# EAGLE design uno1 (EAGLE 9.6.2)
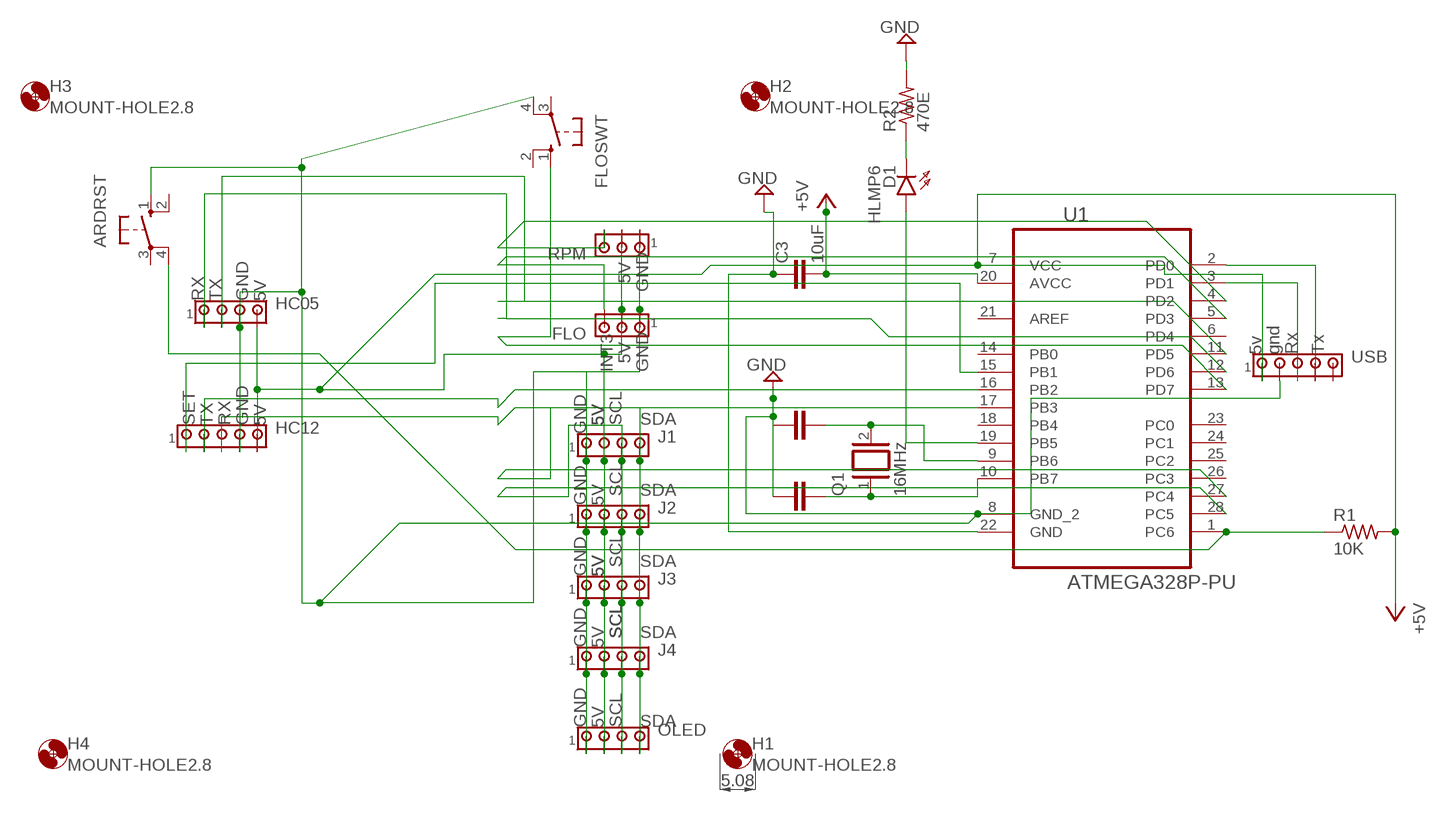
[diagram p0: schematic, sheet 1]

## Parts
ARDRST  10-XX  [B3F-10XX]
C3  10uF  C2.5/2  [C2.5-2]
D1  HLMP6  [HLMP6]
FLO  MTA03-100  [10X03MTA]
FLOSWT  10-XX  [B3F-10XX]
H1  MOUNT-HOLE2.8  [2,8]
H2  MOUNT-HOLE2.8  [2,8]
H3  MOUNT-HOLE2.8  [2,8]
H4  MOUNT-HOLE2.8  [2,8]
HC05  MTA04-100  [10X04MTA]
HC12  MTA05-100  [10X05MTA]
J1  MTA04-100  [10X04MTA]
J2  MTA04-100  [10X04MTA]
J3  MTA04-100  [10X04MTA]
J4  MTA04-100  [10X04MTA]
OLED  MTA04-100  [10X04MTA]
Q1  16MHz  XTAL  [Q]
R1  10K  R-US_0204/5  [0204/5]
R2  470E  R-US_0204/5  [0204/5]
RPM  MTA03-100  [10X03MTA]
U1  ATMEGA328P-PU  [DIP254P762X457-28]
USB  MTA05-100  [10X05MTA]

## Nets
GND: ARDRST.1(S) C3.1 FLO.1 FLOSWT.4(P1) HC05.3 HC12.4 J1.1 J2.1 J3.1 J4.1 OLED.1 R2.2 RPM.1 U1.8(GND_2) U1.22(GND) USB.2
N$1: J1.3 J2.3 J3.3 J4.3 OLED.3 U1.28(PC5)
N$2: J1.4 J2.4 J3.4 J4.4 OLED.4 U1.27(PC4)
N$3: U1.2(PD0) USB.4
N$4: HC12.1 U1.15(PB1)
N$5: U1.3(PD1) USB.3
N$6: FLO.3 U1.5(PD3)
N$7: FLOSWT.1(S) U1.13(PD7)
N$8: HC05.2 U1.11(PD5)
N$9: HC05.1 U1.12(PD6)
N$10: HC12.2 U1.16(PB2)
N$11: HC12.3 U1.17(PB3)
N$13: ARDRST.4(P1) R1.1 U1.1(PC6)
N$14: RPM.3 U1.4(PD2)
N$15: Q1.2 U1.9(PB6)
N$16: Q1.1 U1.10(PB7)
N$21: D1.A U1.19(PB5)
N$22: D1.K R2.1
VCC: C3.2 FLO.2 HC05.4 HC12.5 J1.2 J2.2 J3.2 J4.2 OLED.2 R1.2 RPM.2 U1.7(VCC) U1.20(AVCC) USB.1 ; supply symbol labelled +5V
Unconnected: ARDRST.2(S1) ARDRST.3(P) FLOSWT.2(S1) FLOSWT.3(P) U1.6(PD4) U1.14(PB0) U1.18(PB4) U1.21(AREF) U1.23(PC0) U1.24(PC1) U1.25(PC2) U1.26(PC3) USB.5

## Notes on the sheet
- 5V
- GND
- RX | TX | GND | 5V
- 5v | gnd | Rx | Tx
- 5V
- INT3 | GND
- SET | TX | RX | GND | 5V | 5V | 5V | 5V | SCL | SDA
- GND
- SCL | SDA
- GND | 5V
- SCL | SDA
- GND | 5V | 5V
- SCL | SCL | SCL | SDA
- GND | 5V
- GND | 5V | SCL | SDA

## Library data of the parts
ARDRST FLOSWT = switch-omron:10-XX: OMRON SWITCH; MPN: B3F-1000; OC_FARNELL: 176432; OC_NEWARK: 36M3542
C3 = capacitor-wima:C: CAPACITOR
D1 = display-hp:HLMP6: LED; MF: AGILENT TECHNOLOGIES; MPN: HLMP-6500; OC_FARNELL: 1652490; OC_NEWARK: 40K0088
FLO RPM = con-amp:MTA03-100: AMP connector
H1-H4 = holes:MOUNT-HOLE: MOUNTING HOLE with drill center marker
HC05 J1-J4 OLED = con-amp:MTA04-100: AMP connector
HC12 USB = con-amp:MTA05-100: AMP connector
Q1 = special:XTAL: CRYSTAL
R1 R2 = rcl:R-US_: RESISTOR, American symbol; SPICEPREFIX: R
U1 = Atmel_By_element14_Batch_1-00:ATMEGA328P-PU: 8-bit Microcontroller with In-System Programmable Flash; MPN: ATMEGA328P-PU; OC_FARNELL: 1715487; OC_NEWARK: 15R0268; PACKAGE: PDIP-28; SUPPLIER: Atmel

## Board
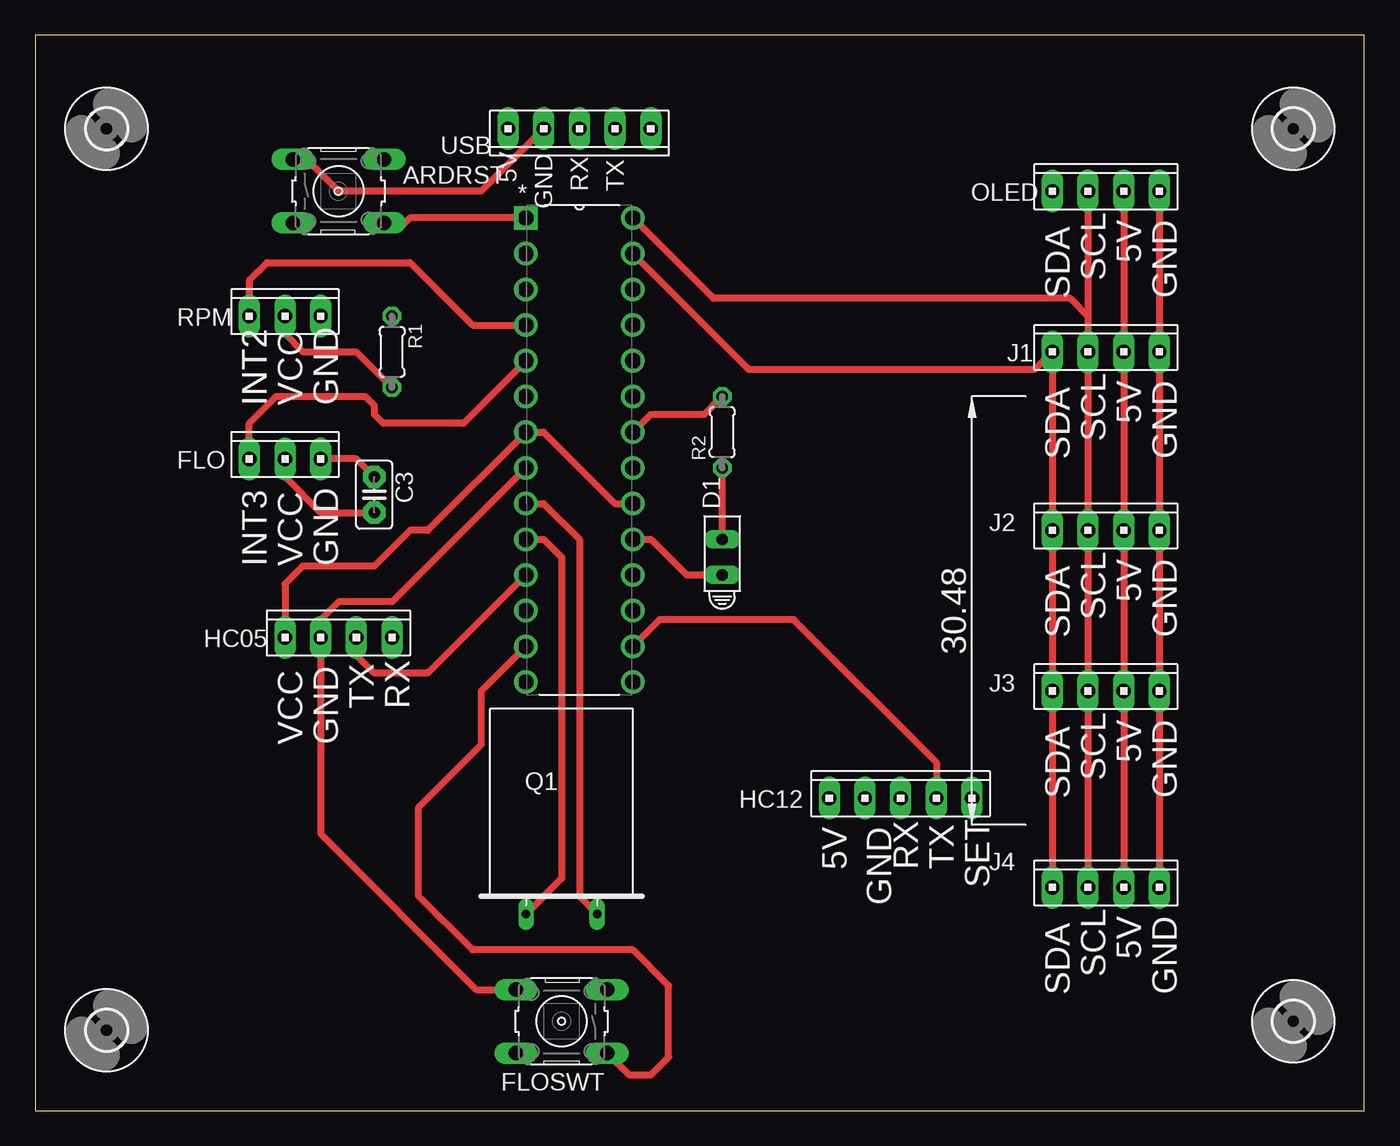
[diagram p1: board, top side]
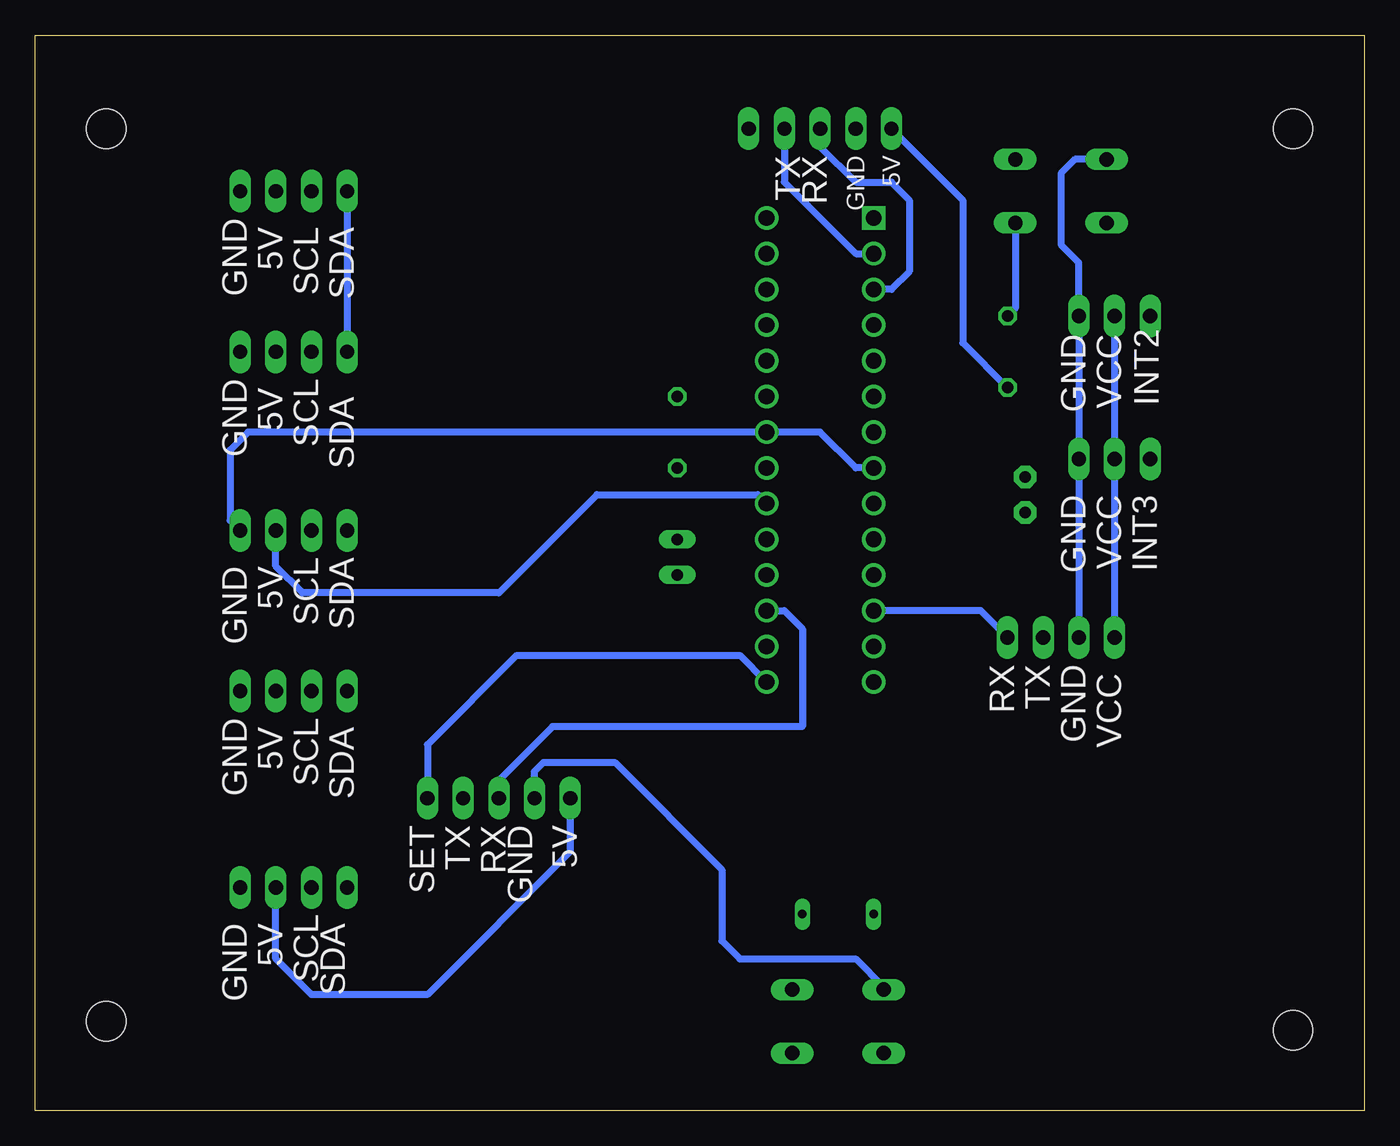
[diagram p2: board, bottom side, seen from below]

Size 94.59 x 76.51 mm. Coordinates in mm from the lower left corner, seen from the top.
Outline: 0,0 94.59,0 94.59,76.51 0,76.51 0,0
Copper layers (1*16): Top 0.035mm / dielectric 1.5mm / Bottom 0.035mm
Design rules "default": minimum track width 6mil, minimum drill 0.35mm, track to track 6mil, track to pad 6mil, pad to pad 6mil, via to via 6mil, smd to smd 6mil, copper to edge 40mil, drill to drill 6mil, minimum pad ring 10mil, minimum via ring 8mil, stop-mask expansion 4mil, vias tented up to drill 0mil, thermal gap 10mil

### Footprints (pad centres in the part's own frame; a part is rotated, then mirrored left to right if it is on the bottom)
B3F-10XX = drill 1.016 long: 1 -3.251,2.261; 2 3.251,2.261; 3 -3.251,-2.261; 4 3.251,-2.261
C2.5-2 = drill 0.813 pad 1.6 octagon: 1 -1.27,0; 2 1.27,0
HLMP6 = drill 0.813 long: A -1.27,0; K 1.27,0
10X03MTA = drill 1.016 long: 1 2.54,0; 2 0,0; 3 -2.54,0
2,8 = hole 2.8: 0,0
10X04MTA = drill 1.016 long: 1 3.81,0; 2 1.27,0; 3 -1.27,0; 4 -3.81,0
10X05MTA = drill 1.016 long: 1 5.08,0; 2 2.54,0; 3 0,0; 4 -2.54,0; 5 -5.08,0
Q = drill 0.61 long: 1 -2.54,-7.62; 2 2.54,-7.62
0204/5 = drill 0.813 octagon: 1 -2.54,0; 2 2.54,0
DIP254P762X457-28 = drill 1.118 square: 1 -7.62,33.02 | drill 1.118: 2 -7.62,30.48; 3 -7.62,27.94; 4 -7.62,25.4; 5 -7.62,22.86; 6 -7.62,20.32; 7 -7.62,17.78; 8 -7.62,15.24; 9 -7.62,12.7; 10 -7.62,10.16; 11 -7.62,7.62; 12 -7.62,5.08; 13 -7.62,2.54; 14 -7.62,0; 15 0,0; 16 0,2.54; 17 0,5.08; 18 0,7.62; 19 0,10.16; 20 0,12.7; 21 0,15.24; 22 0,17.78; 23 0,20.32; 24 0,22.86; 25 0,25.4; 26 0,27.94; 27 0,30.48; 28 0,33.02

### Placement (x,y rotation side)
ARDRST  21.59,65.41 0 top
C3  24.13,43.81 270 top
D1  48.9,39.37 90 top
FLO  17.78,46.35 0 top
FLOSWT  37.46,6.35 180 top
H1  5.08,5.71 0 top
H2  89.53,6.35 0 top
H3  89.53,69.85 0 top
H4  5.08,69.85 0 top
HC05  21.59,33.65 0 top
HC12  61.59,22.23 0 top
J1  76.2,53.97 0 top
J2  76.2,41.27 0 top
J3  76.2,29.84 0 top
J4  76.2,15.88 0 top
OLED  76.2,65.41 0 top
Q1  37.46,21.59 0 top
R1  25.4,53.97 270 top
R2  48.9,48.26 90 top
RPM  17.78,56.51 0 top
U1  42.54,30.48 0 top
USB  38.73,69.85 180 top

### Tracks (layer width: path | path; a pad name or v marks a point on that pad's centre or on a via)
GND
  Top 0.508: J4.1 J3.1 J2.1 J1.1 OLED.1 | FLOSWT.4 31.39,8.61 20.32,19.68 HC05.3 20.32,34.92 21.59,36.2 25.4,36.2 U1.8 | U1.22 43.81,49.53 47.62,49.53 R2.2 | FLO.1 22.86,46.35 C3.1 | ARDRST.1 19.33,67.67 21.59,65.41 31.75,65.41 USB.2
  Bottom 0.508: J2.1 80.72,41.98 80.72,46.99 79.45,48.26 U1.22 38.73,48.26 36.2,45.72 U1.8 | ARDRST.1 20.6,67.67 21.59,66.67 21.59,61.59 20.32,60.32 RPM.1 FLO.1 HC05.3 | HC12.4 59.05,24.13 58.42,24.77 53.34,24.77 45.72,17.14 45.72,12.07 44.45,10.79 36.2,10.79 34.21,8.81 FLOSWT.4
N$1
  Top 0.508: J1.3 J2.3 J3.3 J4.3 | U1.28 48.26,57.78 73.66,57.78 74.93,56.51 J1.3 | OLED.3 J1.3
N$2
  Top 0.508: J4.4 J3.4 J2.4 J1.4 71.12,52.7 50.8,52.7 U1.27
  Bottom 0.508: OLED.4 J1.4
N$3
  Bottom 0.508: USB.4 41.27,66.04 36.2,60.96 U1.2
N$4
  Bottom 0.508: HC12.1 66.67,26.04 60.32,32.38 44.45,32.38 U1.15
N$5
  Bottom 0.508: USB.3 38.73,68.58 36.2,66.04 33.65,66.04 32.38,64.77 32.38,59.69 33.65,58.42 U1.3
N$6
  Top 0.508: FLO.3 15.24,48.89 17.15,50.8 23.49,50.8 24.13,50.16 24.13,49.53 24.76,48.89 30.48,48.89 U1.5
N$7
  Top 0.508: FLOSWT.1 42.27,2.54 43.81,2.54 45.09,3.81 45.09,8.89 42.54,11.43 31.12,11.43 27.3,15.24 27.3,21.59 31.75,26.04 31.75,29.84 U1.13
N$8
  Top 0.508: U1.11 27.94,31.11 24.13,31.11 22.86,32.38 HC05.2
N$9
  Bottom 0.508: HC05.1 27.3,35.56 U1.12
N$10
  Top 0.508: HC12.2 64.13,24.77 53.98,34.92 44.45,34.92 U1.16
N$11
  Bottom 0.508: U1.17 41.27,35.56 40.01,34.29 40.01,27.3 57.79,27.3 61.59,23.5 HC12.3
N$13
  Top 0.508: U1.1 26.67,63.5 26.04,62.87 25.12,62.87 ARDRST.4
  Bottom 0.508: ARDRST.4 24.84,57.07 R1.1
N$14
  Top 0.508: RPM.3 15.24,59.05 16.51,60.32 26.67,60.32 31.12,55.88 U1.4
N$15
  Top 0.508: U1.9 36.2,43.18 38.73,40.64 38.73,15.24 Q1.2
N$16
  Top 0.508: U1.10 36.2,40.64 37.46,39.37 37.46,16.51 Q1.1
N$21
  Top 0.508: U1.19 43.81,40.64 46.35,38.1 D1.A
N$22
  Top 0.508: R2.1 D1.K
VCC
  Top 0.508: J4.2 J3.2 J2.2 J1.2 OLED.2 | FLO.2 17.78,45.08 20.32,42.54 C3.2 | HC05.4 17.78,37.46 19.05,38.73 24.13,38.73 26.67,41.27 27.94,41.27 U1.7 36.2,48.26 41.27,43.18 U1.20 | RPM.2 17.78,55.24 19.05,53.97 22.86,53.97 R1.2
  Bottom 0.508: J2.2 77.47,38.73 75.56,36.83 61.59,36.83 54.61,43.81 43.18,43.81 U1.20 | RPM.2 FLO.2 HC05.4 | J4.2 77.47,10.79 74.93,8.26 66.67,8.26 56.51,18.41 HC12.5 | R1.2 28.57,54.61 28.57,64.77 USB.1

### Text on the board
tPlace: 5V | RX | TX | GND | 5V | SCL | SDA | GND | INT2 | INT2 | VCC | GND | 5V | SCL | SDA | GND | INT3 | VCC | GND | 5V | SCL | SDA | GND | TX | RX | VCC | GND | 5V | SCL | SDA | GND | 5V | RX | TX | SET | GND | 5V | SCL | SDA | GND
bPlace: 5V | GND | RX | TX | GND | SDA | SCL | 5V | VCC | GND | SCL | 5V | GND | SDA | INT2 | INT3 | VCC | GND | SDA | SCL | 5V | GND | GND | TX | RX | VCC | SDA | SCL | 5V | GND | 5V | GND | RX | TX | SET | SDA | SCL | 5V | GND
